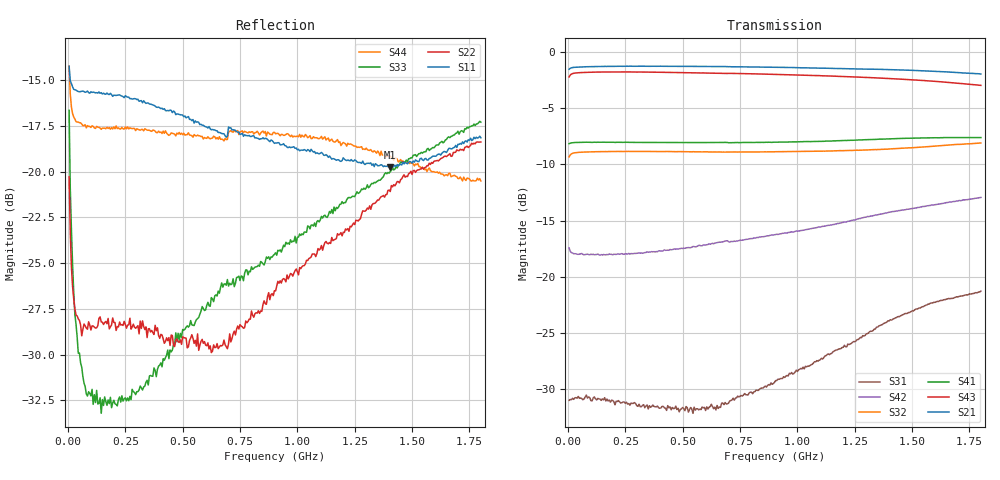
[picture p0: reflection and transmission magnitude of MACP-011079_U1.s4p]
!Agilent Technologies,E5071C,MY46110647,A.11.31
!Date: Tue Nov 07 14:15:35 2023 DD
!Data & Calibration Information:
!MACP-011079 soldered onto PT-0003645 with F connectors, Calibration PT-0003653-TRL. Port1 (pin1) Port2 (pin6) Port3 (pin4) Port4 (pin3)
!Freq	S11:SOLT4(ON)	S12:SOLT4(ON)	S13:SOLT4(ON)	S14:SOLT4(ON)
!	S21:SOLT4(ON)	S22:SOLT4(ON)	S23:SOLT4(ON)	S24:SOLT4(ON)
!	S31:SOLT4(ON)	S32:SOLT4(ON)	S33:SOLT4(ON)	S34:SOLT4(ON)
!	S41:SOLT4(ON)	S42:SOLT4(ON)	S43:SOLT4(ON)	S44:SOLT4(ON)
!PortZ  Port1:75+j0  Port2:75+j0  Port3:75+j0  Port4:75+j0
!Above PortZ is port z conversion or system Z0 setting when saving the data.
!When reading, reference impedance value at option line is always used.
# Hz S MA R 75
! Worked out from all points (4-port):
!   360 points, 5 MHz to 1.8 GHz, reference 75 ohm
!   strongest paths, dB at 5 MHz, 455 MHz, 905 MHz, 1.355 GHz, 1.8 GHz:
!     S21: -1.6, -1.3, -1.4, -1.6, -2.0
!     S43: -2.2, -1.8, -2.0, -2.3, -3.0
!     S41: -8.2, -8.1, -8.0, -7.8, -7.6
!     S32: -9.3, -8.9, -8.9, -8.7, -8.1
!     S42: -17.4, -17.6, -16.2, -14.5, -12.9
!     S31: -31.0, -31.6, -29.2, -24.4, -21.3
!   lowest |S11| = -19.8 dB at 1.405 GHz (marker M1), VSWR 1.23, Z = 62.1 + j5.64 ohm
!   |S11| at or under -10 dB: start of sweep to end of sweep
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5000000  0.1942 161.8  0.8355 4.1  0.03011 25.8  0.3904 -177.5
         0.8359 4.1  0.09677 129.4  0.3408 9.1  0.1347 173.9
         0.02828 25.9  0.3413 9.0  0.147 118.2  0.7736 7.2
         0.3906 -177.5  0.1344 172.6  0.7731 7.3  0.194 150.4
2e7  0.1706 172.9  0.8508 1.1  0.02893 8.1  0.3945 179.6
     0.8506 1.1  0.0486 149.0  0.3538 3.0  0.1279 176.3
     0.02886 7.1  0.3537 3.0  0.05587 119.5  0.7999 1.9
     0.3943 179.6  0.1275 175.8  0.7998 2.0  0.1442 163.8
4.5e7  0.1656 175.4  0.855 -0.2  0.02859 2.7  0.3956 177.4
       0.8551 -0.2  0.0396 169.3  0.3573 1.1  0.1282 176.4
       0.02942 1.7  0.357 1.0  0.03189 126.2  0.8069 -0.3
       0.3958 177.4  0.1259 175.2  0.8071 -0.3  0.1367 167.5
1.45e8  0.1643 174.9  0.8603 -3.1  0.02844 0.7  0.396 170.1
        0.8605 -3.1  0.03883 -172.8  0.36 -1.4  0.1276 171.1
        0.02826 -0.8  0.3598 -1.4  0.02185 122.9  0.8129 -5.0
        0.3964 170.1  0.1256 169.8  0.813 -5.0  0.1305 159.6
6.95e8  0.1251 162.8  0.8588 -17.5  0.02658 17.5  0.3939 132.9
        0.8591 -17.5  0.03281 -122.4  0.3591 -9.8  0.1452 138.1
        0.02728 14.5  0.3584 -9.8  0.05071 39.5  0.8004 -27.4
        0.3954 133.1  0.1446 138.0  0.8009 -27.4  0.1225 97.9
1.405e9  0.1029 154.1  0.8303 -36.4  0.05397 20.3  0.406 86.9
         0.8329 -36.6  0.08824 -126.8  0.3698 -18.1  0.1869 95.1
         0.06443 20.3  0.37 -17.8  0.1001 -7.4  0.7599 -57.1
         0.4105 87.4  0.1939 92.8  0.7597 -57.1  0.1102 55.2
1.8e9  0.1237 142.6  0.7952 -47.6  0.07787 5.6  0.4124 60.6
       0.7967 -47.9  0.1205 -141.6  0.3909 -23.9  0.2205 70.1
       0.0864 4.7  0.3933 -23.7  0.1365 -22.7  0.7097 -75.4
       0.4157 60.7  0.2253 67.2  0.7091 -75.3  0.09432 44.1
